| IBIS file generated by GenIBIS.pl Version 3.22
|   dm385
[IBIS ver]   4.1
[File name]   dm385.ibs
[File Rev]   3.0
[Date]   Tue Oct 30, 2012, 8:51:53
[Source]   Data created at Texas Instruments
[Notes]   CHECKED BY IBISCK4.
   166 warnings can be ignored
   Some pins may contain selectors which are not valid options
   for that particular pin.
   Please refer to the device datasheet for information on picking
   the correct selector model, which depends on various software
   register configurations.
   Some pins are modeled as IO or tri-state for output mode.
[Disclaimer] Please be aware that in the absence of a written agreement,
   Texas Instruments (TI) assumes no liability for: 1) the
   accuracy of the IBIS models provided to your company, 2) the
   proper functioning of these IBIS models in your design or for
   any resulting applications, or, 3) infringement of patents,
   copyrights, or intellectual property rights resulting from
   your use of these IBIS models. TI provides IBIS models as a
   service to our customers and therefore reserves the right to
   limit distribution of the IBIS models.
[Copyright]   Property of Texas Instruments Incorporated. Unauthorised
   reproduction and/or distribution is strictly prohibited. This
   product is protected under copyright law and trade secret law
   as an unpublished work. Created 2010,(C) Copyright 2010,
   Texas Instruments Incorporated., All Rights Reserved. These
   commodities are under the U.S. Government distribution license
   control.As such,they are not to be re-exported without the
   prior approval of the U.S. Department of Commerce.
|   Component dm385
[Component]   dm385
[Manufacturer]   Texas Instruments.
| Source IO level model revisions
|Model   Revision   Date
|BC1833DV40DCPBFBP18LL_SSDHH   1.1   May 27, 2010
|IQ1833DVTCKPBFBP18LL_SSDHH   1.1   May 27, 2010
|BC1833DV50BPBFBP18LL_SSDHV   1.1   May 30, 2010
|IHHV1833DVHYP18LL_SSDHH   1.1   May 27, 2010
|BC1833DV50BPBFBP18LL_SSDHH   1.1   May 30, 2010
|BI2C1833DVFZP18_SSDHH   1.0   May 28, 2010
|BC1833DV40DCPBFBP18LL_SSDHV   1.1   May 27, 2010
|BCSHTLTCSCDVPBFZ_SSDHV   1.0   May 31, 2010
|BCSHTLTCSCDDVPBFZ_SSDHV   1.0   May 31, 2010
[Package]
|   typ   min   max
R_pkg   0.227048417721519   2.87E-2   6.12E-1
L_pkg   1.80481962025317E-009 3.33E-10   4.72E-9
C_pkg   8.93439873417721E-013 5.09E-13   1.66E-12
[Pin]   signal_name   model_name   R_pin   L_pin   C_pin
AF27   AUD_CLKIN1   Selector_5   1.66E-1   1.31E-9   7.51E-13
AG30   AUD_CLKIN2   Selector_5   2.51E-1   2.00E-9   7.85E-13
AF31   AUD_CLKIN0   Selector_5   2.58E-1   2.21E-9   7.02E-13
V30   AUXOSC_MXI   NC
U31   AUXOSC_MXO   NC
AJ31   CLKIN32   Selector_5   3.03E-1   2.21E-9   6.52E-13
AA2   CSI2_DX[2]   NC
V2   CSI2_DY[4]   NC
AC2   CSI2_DY[0]   NC
Y2   CSI2_DY[2]   NC
W2   CSI2_DX[3]   NC
V1   CSI2_DX[4]   NC
W1   CSI2_DY[3]   NC
AA1   CSI2_DX[1]   NC
AB2   CSI2_DX[0]   NC
AB1   CSI2_DY[1]   NC
AL26   DDR[0]_WEN   Selector_9   3.09E-1   2.24E-9   7.45E-13
AJ27   DDR[0]_A[3]   Selector_9   3.09E-1   2.18E-9   9.15E-13
AL23   DDR[0]_A[14]   Selector_9   3.06E-1   2.10E-9   8.49E-13
AK24   DDR[0]_A[11]   Selector_9   3.08E-1   2.21E-9   7.45E-13
AG23   DDR[0]_A[7]   Selector_9   2.86E-1   1.99E-9   1.03E-12
AK9   DDR[0]_D[1]   Selector_8   2.35E-1   1.65E-9   8.84E-13
AJ15   DDR[0]_DQM[2]   Selector_9   2.37E-1   1.45E-9   7.37E-13
AK30   DDR[0]_A[6]   Selector_9   3.09E-1   2.37E-9   8.54E-13
AH23   DDR[0]_A[12]   Selector_9   2.98E-1   2.05E-9   8.52E-13
AL27   DDR[0]_CLK   Selector_9   2.52E-1   2.04E-9   8.22E-13
AH19   DDR[0]_D[26]   Selector_8   2.46E-1   1.65E-9   1.02E-12
AG20   DDR[0]_D[31]   Selector_8   2.57E-1   1.66E-9   1.01E-12
AK29   DDR[0]_A[9]   Selector_9   3.11E-1   2.17E-9   7.34E-13
AC19   DDR[0]_D[29]   Selector_8   1.65E-1   6.79E-10   1.25E-12
AK14   DDR[0]_D[15]   Selector_8   2.56E-1   1.50E-9   8.22E-13
AK13   DDR[0]_D[12]   Selector_8   2.59E-1   1.57E-9   7.06E-13
AK17   DDR[0]_DQS[2]N   Selector_12  2.03E-1   1.95E-9   7.17E-13
AG16   DDR[0]_D[21]   Selector_8   2.33E-1   1.25E-9   8.85E-13
AD15   DDR[0]_D[18]   Selector_8   1.61E-1   1.07E-9   1.03E-12
AC16   DDR[0]_D[23]   Selector_8   1.58E-1   8.32E-10   1.14E-12
AJ23   DDR[0]_A[2]   Selector_9   3.05E-1   2.12E-9   9.93E-13
AL15   DDR[0]_DQS[1]   Selector_12  2.28E-1   1.81E-9   6.85E-13
AG12   DDR[0]_D[9]   Selector_8   2.59E-1   1.32E-9   6.94E-13
AD19   DDR[0]_D[28]   Selector_8   1.70E-1   1.29E-9   1.05E-12
AK15   DDR[0]_DQS[1]N   Selector_12  2.25E-1   1.76E-9   9.52E-13
AJ12   DDR[0]_D[8]   Selector_8   2.60E-1   1.53E-9   8.05E-13
AD12   DDR[0]_D[10]   Selector_8   1.72E-1   7.55E-10   1.03E-12
AL8   DDR[0]_DQM[0]   Selector_9   2.41E-1   1.77E-9   7.77E-13
AJ16   DDR[0]_D[20]   Selector_8   2.33E-1   1.47E-9   7.48E-13
AL12   DDR[0]_D[7]   Selector_8   2.40E-1   1.76E-9   6.73E-13
AL30   DDR[0]_VTP   NC
AL21   DDR[0]_ODT[0]   Selector_9   2.99E-1   2.04E-9   7.45E-13
AL24   DDR[0]_A[0]   Selector_9   3.06E-1   2.36E-9   8.02E-13
AF19   DDR[0]_D[27]   Selector_8   2.32E-1   1.51E-9   9.24E-13
AL20   DDR[0]_DQS[3]   Selector_12  2.23E-1   2.10E-9   8.50E-13
AK22   DDR[0]_A[15]   Selector_9   2.99E-1   2.06E-9   8.71E-13
AK26   DDR[0]_BA[0]   Selector_9   2.88E-1   2.01E-9   8.71E-13
AJ19   DDR[0]_D[25]   Selector_8   2.48E-1   1.87E-9   8.59E-13
AH27   DDR[0]_A[5]   Selector_9   2.90E-1   2.10E-9   8.89E-13
AK25   DDR[0]_CASN   Selector_9   3.10E-1   2.38E-9   8.70E-13
AJ20   DDR[0]_D[30]   Selector_8   2.58E-1   1.54E-9   8.11E-13
AK10   DDR[0]_D[2]   Selector_8   2.34E-1   1.55E-9   7.39E-13
AD23   DDR[0]_A[10]   Selector_9   1.90E-1   1.33E-9   1.10E-12
AD16   DDR[0]_D[22]   Selector_8   1.53E-1   7.63E-10   1.20E-12
AK20   DDR[0]_DQS[3]N   Selector_12  2.20E-1   1.71E-9   7.20E-13
AK16   DDR[0]_D[19]   Selector_8   2.34E-1   2.09E-9   7.88E-13
AJ25   DDR[0]_RASN   Selector_9   3.06E-1   2.36E-9   1.10E-12
AH11   DDR[0]_D[4]   Selector_8   2.36E-1   1.63E-9   1.09E-12
AL14   DDR[0]_D[14]   Selector_8   2.77E-1   2.19E-9   7.20E-13
AL9   DDR[0]_D[0]   Selector_8   2.41E-1   1.84E-9   6.60E-13
AK19   DDR[0]_D[24]   Selector_8   2.63E-1   1.99E-9   8.03E-13
AK27   DDR[0]_CLKN   Selector_9   2.55E-1   1.99E-9   7.91E-13
AJ11   DDR[0]_D[3]   Selector_8   2.28E-1   1.48E-9   7.79E-13
AC22   DDR[0]_A[1]   Selector_9   1.99E-1   1.56E-9   1.21E-12
AK28   DDR[0]_A[4]   Selector_9   3.07E-1   2.35E-9   9.20E-13
AF23   DDR[0]_BA[1]   Selector_9   2.79E-1   1.74E-9   9.46E-13
AK18   DDR[0]_DQM[3]   Selector_9   2.62E-1   1.71E-9   7.74E-13
AK11   DDR[0]_DQS[0]N   Selector_12  1.97E-1   1.57E-9   7.59E-13
AK12   DDR[0]_DQM[1]   Selector_9   2.61E-1   1.73E-9   6.87E-13
AB21   DDR[0]_CS[0]N   Selector_9   1.89E-1   1.60E-9   1.21E-12
AH15   DDR[0]_D[16]   Selector_8   2.32E-1   1.43E-9   7.75E-13
AL17   DDR[0]_DQS[2]   Selector_12  2.06E-1   2.04E-9   6.57E-13
AF15   DDR[0]_D[17]   Selector_8   2.33E-1   1.25E-9   7.62E-13
AD9   DDR[0]_D[5]   Selector_8   1.50E-1   1.11E-9   1.08E-12
AF11   DDR[0]_D[6]   Selector_8   2.23E-1   1.41E-9   7.17E-13
AL29   DDR[0]_A[8]   Selector_9   3.11E-1   2.25E-9   8.11E-13
AC13   DDR[0]_D[13]   Selector_8   1.77E-1   9.38E-10   7.90E-13
AA20   DDR[0]_RST   Selector_9   1.14E-1   1.28E-9   1.23E-12
AD20   DDR[0]_CKE   Selector_9   1.85E-1   1.25E-9   1.14E-12
AL11   DDR[0]_DQS[0]   Selector_12  2.00E-1   1.74E-9   8.08E-13
AK23   DDR[0]_A[13]   Selector_9   3.07E-1   2.17E-9   9.86E-13
AH25   DDR[0]_BA[2]   Selector_9   2.98E-1   2.18E-9   1.24E-12
AB12   DDR[0]_D[11]   Selector_8   1.92E-1   9.34E-10   1.25E-12
F30   DEVOSC_MXI   NC
G31   DEVOSC_MXO   NC
U28   DEVOSC_WAKE   Selector_5   1.35E-1   1.20E-9   7.62E-13
AH1   EMAC[0]_MCOL   Selector_5   3.85E-1   2.94E-9   9.55E-13
AL3   EMAC[0]_MRXD[2]   Selector_5   3.82E-1   2.76E-9   1.06E-12
AH8   EMAC[0]_MTXD[6]   Selector_5   1.63E-1   1.30E-9   7.04E-13
AJ6   EMAC[0]_MRXDV   Selector_5   2.42E-1   1.83E-9   7.69E-13
AJ2   EMAC[0]_MRXER   Selector_5   3.56E-1   2.48E-9   9.44E-13
AE4   EMAC[0]_MTXD[3]   Selector_5   1.06E-1   1.05E-9   9.05E-13
AG1   EMAC_RMREFCLK   Selector_5   3.61E-1   2.77E-9   1.09E-12
AK7   EMAC[0]_MTXD[2]   Selector_5   2.54E-1   2.10E-9   9.24E-13
AL5   EMAC[0]_MRXD[6]   Selector_5   3.30E-1   2.32E-9   9.10E-13
AK4   EMAC[0]_MRXD[4]   Selector_5   3.22E-1   2.36E-9   1.06E-12
AK3   EMAC[0]_MRXD[3]   Selector_5   3.32E-1   2.46E-9   1.18E-12
AK6   EMAC[0]_MTXD[0]   Selector_5   2.62E-1   2.01E-9   9.37E-13
AL6   EMAC[0]_GMTCLK   Selector_5   3.33E-1   2.48E-9   9.02E-13
AJ7   EMAC[0]_MTXD[1]   Selector_5   2.29E-1   1.79E-9   9.75E-13
AK5   EMAC[0]_MRXD[7]   Selector_5   2.92E-1   2.07E-9   1.01E-12
AJ8   EMAC[0]_MTXD[5]   Selector_5   2.05E-1   1.57E-9   7.51E-13
AF8   EMAC[0]_MTXEN   Selector_5   4.94E-2   5.14E-10   6.62E-13
AH2   EMAC[0]_MCRS   Selector_5   3.49E-1   2.48E-9   1.18E-12
AG4   EMAC[0]_MTCLK   Selector_5   2.64E-1   1.97E-9   1.04E-12
AK1   EMAC[0]_MRCLK   Selector_5   4.24E-1   2.94E-9   1.10E-12
AK8   EMAC[0]_MTXD[4]   Selector_5   2.39E-1   1.84E-9   9.63E-13
AL2   EMAC[0]_MRXD[1]   Selector_5   4.00E-1   2.78E-9   1.05E-12
AG8   EMAC[0]_MTXD[7]   Selector_5   9.95E-2   7.49E-10   7.36E-13
AJ4   EMAC[0]_MRXD[5]   Selector_5   2.84E-1   2.10E-9   9.81E-13
AK2   EMAC[0]_MRXD[0]   Selector_5   3.75E-1   2.65E-9   1.01E-12
A18   EMU0   Selector_16  2.53E-1   2.14E-9   6.98E-13
B19   EMU1   Selector_16  2.48E-1   1.95E-9   8.34E-13
R2   GPMC_D[13]   Selector_5   2.29E-1   1.71E-9   5.72E-13
AA10   GPMC_ADVN_ALE   Selector_5   1.88E-1   1.72E-9   1.00E-12
M2   GPMC_A[17]   Selector_5   2.33E-1   1.87E-9   7.47E-13
M1   GPMC_A[16]   Selector_5   2.62E-1   2.35E-9   5.77E-13
M3   GPMC_A[18]   Selector_5   2.04E-1   1.56E-9   8.46E-13
T8   GPMC_D[9]   Selector_5   4.04E-2   4.40E-10   7.71E-13
T1   GPMC_D[8]   Selector_5   2.67E-1   2.02E-9   6.50E-13
W6   GPMC_D[0]   Selector_5   1.30E-1   1.38E-9   1.04E-12
N9   GPMC_A[20]   Selector_5   3.84E-2   4.90E-10   7.79E-13
M5   GPMC_A[19]   Selector_5   1.34E-1   1.21E-9   7.39E-13
T3   GPMC_D[6]   Selector_5   1.90E-1   1.37E-9   7.92E-13
W9   GPMC_D[4]   Selector_5   9.55E-2   1.25E-9   1.07E-12
N1   GPMC_A[21]   Selector_5   2.61E-1   1.95E-9   5.85E-13
AB9   GPMC_CLK   Selector_5   2.06E-1   1.80E-9   1.13E-12
N2   GPMC_A[22]   Selector_5   2.29E-1   1.70E-9   7.54E-13
Y5   GPMC_WEN   Selector_5   1.86E-1   1.70E-9   1.05E-12
R1   GPMC_D[14]   Selector_5   2.65E-1   1.82E-9   6.57E-13
R6   GPMC_D[10]   Selector_5   9.06E-2   7.90E-10   7.40E-13
W8   GPMC_WAIT[0]   Selector_5   7.07E-2   9.84E-10   1.05E-12
Y3   GPMC_BE[0]N_CLE   Selector_5   2.26E-1   2.44E-9   8.93E-13
AC9   GPMC_CS[0]N   Selector_5   2.25E-1   1.92E-9   1.34E-12
P2   GPMC_D[15]   Selector_5   2.07E-1   1.56E-9   6.41E-13
W4   GPMC_D[1]   Selector_5   1.69E-1   1.62E-9   8.93E-13
Y8   GPMC_OE_REN   Selector_5   8.78E-2   1.18E-9   1.09E-12
AC3   GPMC_CS[2]N   Selector_5   2.27E-1   1.79E-9   7.80E-13
T5   GPMC_D[5]   Selector_5   1.08E-1   1.05E-9   7.69E-13
AG6   GPMC_CS[4]N   Selector_5   2.47E-1   2.00E-9   1.10E-12
W3   GPMC_D[2]   Selector_5   2.21E-1   1.94E-9   8.39E-13
R3   GPMC_D[12]   Selector_5   1.81E-1   1.43E-9   6.41E-13
AA12   GPMC_CS[1]N   Selector_5   1.16E-1   1.42E-9   1.27E-12
T2   GPMC_D[7]   Selector_5   2.27E-1   1.73E-9   6.57E-13
AF2   GPMC_CS[3]N   Selector_5   3.08E-1   2.32E-9   9.30E-13
R8   GPMC_A[23]   Selector_5   3.63E-2   3.74E-10   7.91E-13
U2   GPMC_D[3]   Selector_5   2.06E-1   1.77E-9   8.63E-13
Y11   GPMC_BE[1]N   Selector_5   1.65E-1   1.70E-9   1.27E-12
R4   GPMC_D[11]   Selector_5   1.33E-1   1.15E-9   7.09E-13
A9   HDDAC_A   NC
B7   HDDAC_VREF   NC
B6   HDDAC_IREF   NC
E9   HDDAC_HSYNC   Selector_4   6.43E-2   5.68E-10   6.01E-13
A8   HDDAC_B   NC
D9   HDDAC_VSYNC   Selector_4   9.70E-2   9.00E-10   8.07E-13
B8   HDDAC_C   NC
A15   HDMI_CLKP   NC
A12   HDMI_DN2   NC
B13   HDMI_DN1   NC
A14   HDMI_DN0   NC
B14   HDMI_DP0   NC
B15   HDMI_CLKN   NC
A11   HDMI_DP2   NC
B12   HDMI_DP1   NC
D2   I2C[1]_SCL   Selector_2   3.52E-1   2.57E-9   1.14E-12
T24   I2C[0]_SDA   Selector_2   3.75E-2   3.33E-10   9.91E-13
T27   I2C[0]_SCL   Selector_2   1.10E-1   9.87E-10   6.35E-13
D1   I2C[1]_SDA   Selector_2   3.78E-1   2.72E-9   8.43E-13
Y21   MCA[1]_AXR[1]   Selector_14  8.08E-2   9.66E-10   1.38E-12
AC24   MCA[1]_AFSR   Selector_14  5.51E-2   6.17E-10   8.58E-13
AD29   MCA[1]_ACLKR   Selector_14  1.99E-1   1.54E-9   7.47E-13
AD30   MCA[0]_ACLKR   Selector_14  2.42E-1   1.99E-9   6.99E-13
AF29   MCA[0]_AXR[0]   Selector_14  2.04E-1   1.55E-9   6.97E-13
AC31   MCA[0]_AXR[3]   Selector_14  2.55E-1   1.97E-9   7.06E-13
AE31   MCA[0]_AXR[1]   Selector_14  2.49E-1   1.80E-9   6.83E-13
Y22   MCA[1]_AXR[0]   Selector_14  4.32E-2   7.12E-10   9.06E-13
AC23   MCA[1]_ACLKX   Selector_14  6.51E-2   7.77E-10   9.32E-13
AD27   MCA[0]_AXR[5]   Selector_14  1.30E-1   1.24E-9   8.34E-13
AD28   MCA[0]_ACLKX   Selector_14  1.42E-1   1.50E-9   6.83E-13
AD26   MCA[0]_AXR[4]   Selector_14  1.05E-1   1.03E-9   7.96E-13
AE30   MCA[0]_AXR[2]   Selector_14  2.22E-1   1.81E-9   7.42E-13
AB22   MCA[1]_AFSX   Selector_14  5.70E-2   5.46E-10   9.60E-13
AE29   MCA[0]_AFSX   Selector_14  1.74E-1   1.70E-9   7.57E-13
AF30   MCA[0]_AFSR   Selector_14  2.24E-1   1.87E-9   7.37E-13
AG2   MDCLK   Selector_5   3.17E-1   2.33E-9   9.92E-13
AG3   MDIO   Selector_5   2.95E-1   2.33E-9   8.47E-13
AH31   NMIN   Selector_7   3.08E-1   2.07E-9   8.90E-13
K31   PCIE_TXN0   NC
K30   PCIE_RXP0   NC
L31   PCIE_TXP0   NC
J30   PCIE_RXN0   NC
AH30   PORN   Selector_6   2.59E-1   1.86E-9   9.14E-13
AH29   RESETN   Selector_7   2.35E-1   1.62E-9   6.89E-13
AJ30   RSTOUT_WD_OUTN   Selector_10  2.70E-1   1.93E-9   9.49E-13
J25   RSV0   NC
H24   RSV2   NC
H28   RSV3   NC
L30   RSV27   NC
M30   RSV28   NC
N30   RSV29   NC
N31   RSV30   NC
P31   RSV31   NC
R30   RSV32   NC
T30   RSV33   NC
AK21   RSV42   Selector_9   2.98E-1   1.94E-9   9.19E-13
P30   RSV43   NC
N29   RTCK   Selector_13  1.55E-1   1.58E-9   8.66E-13
AB31   SD0_DAT[6]   Selector_14  2.34E-1   1.97E-9   7.86E-13
AC30   SD0_DAT[7]   Selector_14  2.32E-1   1.88E-9   8.26E-13
AB30   SD0_CLK   Selector_5   2.14E-1   1.76E-9   6.98E-13
Y30   SD0_DAT[3]   Selector_5   1.93E-1   1.62E-9   7.33E-13
AA28   SD0_DAT[0]   Selector_5   1.42E-1   1.34E-9   7.40E-13
AA26   SD0_DAT[1]_SDIRQN   Selector_5   9.56E-2   1.03E-9   8.42E-13
Y31   SD0_DAT[2]_SDRWN   Selector_5   2.25E-1   1.96E-9   7.06E-13
AA29   SD0_CMD   Selector_5   1.70E-1   1.55E-9   7.83E-13
AA30   SD1_DAT[1]_SDIRQN   Selector_5   2.74E-1   2.10E-9   8.23E-13
W31   SD1_DAT[0]   Selector_5   2.51E-1   1.84E-9   7.39E-13
W30   SD1_CLK   Selector_4   2.00E-1   1.61E-9   7.96E-13
Y27   SD1_DAT[3]   Selector_5   1.24E-1   1.16E-9   8.87E-13
Y29   SD1_CMD   Selector_5   1.83E-1   1.49E-9   8.27E-13
U29   SD1_DAT[2]_SDRWN   Selector_5   1.62E-1   1.41E-9   6.87E-13
AE3   SD2_DAT[7]   Selector_5   2.41E-1   1.84E-9   9.36E-13
AC6   SD2_SCLK   Selector_5   1.65E-1   1.48E-9   8.89E-13
AC8   SD2_DAT[2]_SDRWN   Selector_5   1.27E-1   1.10E-9   1.08E-12
AC4   SD2_DAT[0]   Selector_5   1.93E-1   1.54E-9   7.61E-13
AC5   SD2_DAT[1]_SDIRQN   Selector_5   1.79E-1   1.54E-9   8.62E-13
AD2   SD2_DAT[4]   Selector_5   2.68E-1   2.16E-9   9.23E-13
AD1   SD2_DAT[3]   Selector_5   3.11E-1   2.59E-9   6.39E-13
AE2   SD2_DAT[6]   Selector_5   2.66E-1   2.13E-9   6.74E-13
AE1   SD2_DAT[5]   Selector_5   3.04E-1   2.41E-9   8.36E-13
H31   SERDES_CLKN   NC
H30   SERDES_CLKP   NC
N23   SPI[1]_D[0]   Selector_11  6.99E-2   6.82E-10   1.09E-12
J28   SPI[0]_D[0]   Selector_11  1.42E-1   1.36E-9   8.74E-13
M29   SPI[1]_SCLK   Selector_11  1.51E-1   1.45E-9   8.33E-13
N24   SPI[0]_SCLK   Selector_16  1.14E-1   1.30E-9   1.22E-12
G28   SPI[0]_SCS[1]N   Selector_11  1.77E-1   1.43E-9   7.49E-13
J27   SPI[0]_D[1]   Selector_11  1.16E-1   1.07E-9   6.17E-13
J29   SPI[1]_SCS[0]N   Selector_11  1.53E-1   1.56E-9   6.76E-13
G29   SPI[0]_SCS[0]N   Selector_11  1.88E-1   1.53E-9   7.64E-13
M27   SPI[1]_D[1]   Selector_11  9.96E-2   1.02E-9   7.76E-13
T29   TCLK   Selector_15  1.55E-1   1.39E-9   7.00E-13
N28   TDI   Selector_3   1.49E-1   1.31E-9   8.10E-13
U26   TDO   Selector_4   8.14E-2   8.38E-10   6.47E-13
T31   TMS   Selector_7   2.63E-1   2.02E-9   6.65E-13
U24   TRSTN   Selector_7   3.68E-2   3.94E-10   7.07E-13
B10   TV_VFB0   NC
B11   TV_RSET   NC
B9   TV_OUT0   NC
E30   UART0_DTRN   Selector_11  2.32E-1   1.69E-9   7.42E-13
J26   UART0_RXD   Selector_3   5.32E-2   5.77E-10   6.66E-13
E29   UART0_DSRN   Selector_11  2.20E-1   1.69E-9   7.10E-13
E28   UART0_TXD   Selector_1   1.93E-1   1.74E-9   9.07E-13
N26   UART0_RIN   Selector_11  1.22E-1   1.26E-9   7.65E-13
D31   UART0_RTSN   Selector_11  2.94E-1   2.30E-9   9.20E-13
D30   UART0_CTSN   Selector_11  2.65E-1   2.20E-9   8.68E-13
E31   UART0_DCDN   Selector_11  2.75E-1   2.23E-9   8.81E-13
L22   UART2_RXD   Selector_11  1.11E-1   1.13E-9   1.58E-12
M21   UART2_TXD   Selector_11  1.42E-1   1.48E-9   1.66E-12
A21   USB0_DP   NC
A20   USB0_ID   NC
B22   USB0_VBUSIN   NC
B20   USB0_CE   NC
B21   USB0_DM   NC
K23   USB0_DRVVBUS   Selector_11  1.02E-1   1.05E-9   1.20E-12
A23   USB1_DP   NC
A24   USB1_ID   NC
C21   USB1_CE   NC
B24   USB1_VBUSIN   NC
B23   USB1_DM   NC
D17   VIN[0]A_D[4]   Selector_11  1.46E-1   1.34E-9   7.23E-13
H16   VIN[0]A_D[13]_BD[5]  Selector_16  4.14E-2   5.78E-10   8.16E-13
L20   VIN[0]A_D[6]   Selector_11  2.11E-1   1.81E-9   1.09E-12
D13   VIN[0]A_HSYNC   Selector_11  1.73E-1   1.98E-9   8.59E-13
C9   VIN[0]A_CLK   Selector_11  1.40E-1   1.69E-9   7.74E-13
K11   VIN[0]A_D[16]   Selector_5   1.34E-1   1.26E-9   1.25E-12
B18   VIN[0]A_D[0]   Selector_11  2.31E-1   1.90E-9   7.19E-13
B16   VIN[0]A_D[8]_BD[0]   Selector_11  2.10E-1   1.77E-9   5.77E-13
B5   VIN[0]A_DE1   Selector_5   2.78E-1   1.92E-9   8.57E-13
A6   VIN[0]A_D[22]   Selector_5   2.74E-1   2.02E-9   6.72E-13
C13   VIN[0]A_VSYNC   Selector_11  2.01E-1   2.09E-9   8.83E-13
J16   VIN[0]A_D[12]_BD[4]  Selector_16  4.57E-2   8.08E-10   9.63E-13
H20   VIN[0]A_D[7]   Selector_11  1.44E-1   1.76E-9   1.03E-12
F17   VIN[0]A_D[5]   Selector_11  7.66E-2   8.46E-10   8.35E-13
A17   VIN[0]A_D[1]   Selector_11  2.54E-1   2.21E-9   5.62E-13
F13   VIN[0]A_D[14]_BD[6]  Selector_16  1.19E-1   1.18E-9   7.73E-13
C7   VIN[0]A_D[21]   Selector_5   1.72E-1   1.61E-9   7.09E-13
C12   VIN[0]A_DE   Selector_16  1.85E-1   1.77E-9   7.90E-13
H13   VIN[0]A_D[15]_BD[7]  Selector_16  3.45E-2   5.26E-10   1.05E-12
K10   VIN[0]A_D[18]   Selector_5   1.04E-1   1.29E-9   1.15E-12
H12   VIN[0]B_CLK   Selector_16  9.56E-2   7.63E-10   9.70E-13
E12   VIN[0]A_D[17]   Selector_5   1.39E-1   1.57E-9   8.57E-13
C16   VIN[0]A_D[9]_BD[1]   Selector_16  1.76E-1   1.36E-9   6.41E-13
F9   VIN[0]A_D[20]   Selector_5   5.09E-2   5.93E-10   6.53E-13
E16   VIN[0]A_D[10]_BD[2]  Selector_16  1.07E-1   9.58E-10   7.96E-13
C17   VIN[0]A_D[3]   Selector_11  1.94E-1   1.67E-9   7.64E-13
H17   VIN[0]A_D[11]_BD[3]  Selector_16  6.05E-2   7.18E-10   9.63E-13
J13   VIN[0]A_FLD   Selector_16  1.19E-1   1.15E-9   9.81E-13
A5   VIN[0]A_D[23]   Selector_5   2.65E-1   1.94E-9   8.01E-13
B17   VIN[0]A_D[2]   Selector_11  2.09E-1   1.89E-9   6.48E-13
D7   VIN[0]A_D[19]   Selector_5   1.24E-1   1.23E-9   7.02E-13
A3   VIN[0]B_FLD   Selector_5   3.26E-1   2.44E-9   9.24E-13
C5   VIN[0]B_DE   Selector_5   2.54E-1   1.79E-9   8.45E-13
B4   VIN[0]A_FLD1   Selector_5   2.78E-1   1.97E-9   8.74E-13
L3   VOUT[1]_G_Y_YC[8]   Selector_5   1.66E-1   1.32E-9   7.96E-13
B27   VOUT[0]_G_Y_YC[8]   Selector_13  4.86E-1   4.13E-9   1.00E-12
C25   VOUT[0]_G_Y_YC[2]   Selector_16  4.92E-1   4.09E-9   1.09E-12
L2   VOUT[1]_G_Y_YC[2]   Selector_5   2.34E-1   1.94E-9   7.55E-13
D5   VOUT[1]_B_CB_C[1]   Selector_5   2.40E-1   1.73E-9   8.85E-13
J1   VOUT[1]_G_Y_YC[5]   Selector_5   3.03E-1   2.19E-9   6.15E-13
E2   VOUT[1]_HSYNC   Selector_5   3.24E-1   2.34E-9   7.87E-13
K2   VOUT[1]_R_CR[9]   Selector_5   2.39E-1   1.90E-9   8.14E-13
B25   VOUT[0]_G_Y_YC[7]   Selector_13  4.43E-1   3.16E-9   1.06E-12
B3   VOUT[0]_FLD   Selector_5   3.12E-1   2.30E-9   9.13E-13
D21   VOUT[0]_B_CB_C[3]   Selector_16  2.22E-1   2.02E-9   9.46E-13
B28   VOUT[0]_R_CR[3]   Selector_16  5.48E-1   4.52E-9   1.20E-12
F21   VOUT[0]_HSYNC   Selector_13  1.58E-1   1.50E-9   1.09E-12
H6   VOUT[1]_G_Y_YC[3]   Selector_5   1.73E-1   1.53E-9   8.12E-13
J10   VOUT[1]_FLD   Selector_5   4.39E-2   7.65E-10   1.05E-12
F24   VOUT[0]_B_CB_C[2]   Selector_16  2.33E-1   2.01E-9   1.10E-12
A26   VOUT[0]_G_Y_YC[6]   Selector_13  4.67E-1   3.58E-9   1.07E-12
J2   VOUT[1]_R_CR[8]   Selector_5   2.25E-1   1.83E-9   7.52E-13
G1   VOUT[1]_B_CB_C[5]   Selector_5   3.30E-1   2.54E-9   8.23E-13
K22   VOUT[0]_CLK   Selector_13  1.58E-1   2.10E-9   1.06E-12
L4   VOUT[1]_R_CR[3]   Selector_5   1.64E-1   1.39E-9   5.09E-13
E24   VOUT[0]_B_CB_C[7]   Selector_13  2.56E-1   2.41E-9   1.19E-12
L6   VOUT[1]_R_CR[2]   Selector_5   8.86E-2   9.28E-10   8.58E-13
L12   VOUT[1]_R_CR[6]   Selector_5   6.32E-2   9.24E-10   1.37E-12
A30   VOUT[0]_R_CR[8]   Selector_13  6.12E-1   4.47E-9   1.23E-12
B29   VOUT[0]_R_CR[4]   Selector_13  5.47E-1   3.88E-9   1.38E-12
J9   VOUT[1]_G_Y_YC[7]   Selector_5   1.45E-1   1.37E-9   1.11E-12
C20   VOUT[0]_AVID   Selector_16  2.07E-1   2.09E-9   7.79E-13
H3   VOUT[1]_B_CB_C[7]   Selector_5   2.41E-1   1.81E-9   9.03E-13
C26   VOUT[0]_G_Y_YC[3]   Selector_16  5.42E-1   4.48E-9   1.33E-12
M11   VOUT[1]_R_CR[5]   Selector_5   6.82E-2   9.06E-10   1.32E-12
J23   VOUT[0]_B_CB_C[4]   Selector_13  1.55E-1   1.92E-9   1.32E-12
H9   VOUT[1]_B_CB_C[0]   Selector_5   6.96E-2   8.39E-10   7.72E-13
H2   VOUT[1]_R_CR[4]   Selector_5   3.39E-1   2.98E-9   8.40E-13
B26   VOUT[0]_G_Y_YC[5]   Selector_13  4.86E-1   3.78E-9   1.23E-12
E26   VOUT[0]_G_Y_YC[4]   Selector_13  5.53E-1   4.72E-9   1.56E-12
B31   VOUT[0]_R_CR[9]   Selector_13  6.11E-1   4.51E-9   1.27E-12
A29   VOUT[0]_R_CR[5]   Selector_13  5.79E-1   4.17E-9   1.15E-12
A27   VOUT[0]_G_Y_YC[9]   Selector_13  5.11E-1   4.30E-9   1.04E-12
J8   VOUT[1]_G_Y_YC[4]   Selector_5   1.17E-1   1.09E-9   6.74E-13
D24   VOUT[0]_B_CB_C[8]   Selector_13  2.72E-1   2.61E-9   1.22E-12
C30   VOUT[0]_R_CR[6]   Selector_13  5.56E-1   4.08E-9   1.51E-12
C2   VOUT[1]_R_CR[0]   Selector_5   3.73E-1   2.49E-9   9.34E-13
F3   VOUT[1]_B_CB_C[4]   Selector_5   2.86E-1   2.02E-9   8.63E-13
J24   VOUT[0]_B_CB_C[6]   Selector_13  2.73E-1   2.62E-9   1.30E-12
G2   VOUT[1]_B_CB_C[6]   Selector_5   2.99E-1   2.35E-9   7.67E-13
F5   VOUT[1]_VSYNC   Selector_5   2.31E-1   1.67E-9   1.03E-12
C24   VOUT[0]_B_CB_C[9]   Selector_13  2.95E-1   2.80E-9   1.02E-12
H5   VOUT[1]_B_CB_C[9]   Selector_5   2.12E-1   1.73E-9   1.03E-12
M8   VOUT[1]_B_CB_C[2]   Selector_5   2.87E-2   4.25E-10   7.42E-13
C28   VOUT[0]_R_CR[2]   Selector_16  5.31E-1   3.97E-9   1.39E-12
G3   VOUT[1]_B_CB_C[8]   Selector_5   2.72E-1   2.26E-9   8.65E-13
B30   VOUT[0]_R_CR[7]   Selector_13  5.89E-1   4.20E-9   1.37E-12
F2   VOUT[1]_B_CB_C[3]   Selector_5   3.10E-1   2.28E-9   9.84E-13
F1   VOUT[1]_AVID   Selector_5   3.29E-1   2.44E-9   7.25E-13
A2   VOUT[1]_G_Y_YC[1]   Selector_5   3.72E-1   2.89E-9   9.50E-13
C1   VOUT[1]_R_CR[1]   Selector_5   3.93E-1   2.74E-9   8.47E-13
B2   VOUT[1]_G_Y_YC[0]   Selector_5   3.58E-1   2.54E-9   1.08E-12
H23   VOUT[0]_B_CB_C[5]   Selector_13  1.44E-1   1.58E-9   9.40E-13
K1   VOUT[1]_G_Y_YC[9]   Selector_5   2.77E-1   2.16E-9   7.40E-13
H4   VOUT[1]_G_Y_YC[6]   Selector_5   2.16E-1   1.61E-9   9.62E-13
E20   VOUT[0]_VSYNC   Selector_13  1.60E-1   1.53E-9   1.02E-12
M10   VOUT[1]_R_CR[7]   Selector_5   4.38E-2   5.27E-10   7.99E-13
D3   VOUT[1]_CLK   Selector_5   3.17E-1   2.20E-9   6.90E-13
AL18   VREFSSTL_DDR[0]   NC
U30   VSSA_AUXOSC   NC
G30   VSSA_DEVOSC   NC
[Diff Pin]   inv_pin   vdiff   tdelay_typ
|DDR[0]_DQS[3]   DDR[0]_DQS[3]N
AL20   AK20   200m   NA
|DDR[0]_DQS[2]   DDR[0]_DQS[2]N
AL17   AK17   200m   NA
|DDR[0]_DQS[1]   DDR[0]_DQS[1]N
AL15   AK15   200m   NA
|DDR[0]_DQS[0]   DDR[0]_DQS[0]N
AL11   AK11   200m   NA
|   Usage OUTPUT#1.8/3.3#X#X#BC1833DV50BPBFBP18LL_SSDHV.PAD
|   Base model BC1833DV50BPBFBP18LL_SSDHV
[Model Selector] Selector_1
Model_37 I/O,1.8V,Pull-down,NORMAL,IND,5%
Model_38 I/O,1.8V,Pull-up,NORMAL,IND,5%
Model_39 I/O,1.8V,Pull-up/down off,NORMAL,IND,5%
Model_40 I/O,3.3V,Pull-down,NORMAL,IND,5%
Model_41 I/O,3.3V,Pull-up,NORMAL,IND,5%
Model_42 I/O,3.3V,Pull-up/down off,NORMAL,IND,5%
Model_43 I/O,1.8V,Pull-down,NORMAL,IND,10%
Model_44 I/O,1.8V,Pull-up,NORMAL,IND,10%
Model_45 I/O,1.8V,Pull-up/down off,NORMAL,IND,10%
Model_46 I/O,3.3V,Pull-down,NORMAL,IND,10%
Model_47 I/O,3.3V,Pull-up,NORMAL,IND,10%
Model_48 I/O,3.3V,Pull-up/down off,NORMAL,IND,10%
|   Usage I/O#1.8/3.3#X#X#BI2C1833DVFZP18_SSDHH.PAD
|   Base model BI2C1833DVFZP18_SSDHH
[Model Selector] Selector_2
Model_65 I/O_OPEN_DRAIN,1.8V,NORMAL,I2C STANDARD,IND,5%
Model_66 I/O_OPEN_DRAIN,3.3V,NORMAL,I2C STANDARD,IND,5%
Model_67 I/O_OPEN_DRAIN,1.8V,NORMAL,I2C STANDARD,IND,10%
Model_68 I/O_OPEN_DRAIN,3.3V,NORMAL,I2C STANDARD,IND,10%
|   Usage INPUT#1.8/3.3#X#X#BC1833DV50BPBFBP18LL_SSDHV.PAD
|   Base model BC1833DV50BPBFBP18LL_SSDHV
[Model Selector] Selector_3
Model_37 I/O,1.8V,Pull-down,NORMAL,IND,5%
Model_38 I/O,1.8V,Pull-up,NORMAL,IND,5%
Model_39 I/O,1.8V,Pull-up/down off,NORMAL,IND,5%
Model_40 I/O,3.3V,Pull-down,NORMAL,IND,5%
Model_41 I/O,3.3V,Pull-up,NORMAL,IND,5%
Model_42 I/O,3.3V,Pull-up/down off,NORMAL,IND,5%
Model_43 I/O,1.8V,Pull-down,NORMAL,IND,10%
Model_44 I/O,1.8V,Pull-up,NORMAL,IND,10%
Model_45 I/O,1.8V,Pull-up/down off,NORMAL,IND,10%
Model_46 I/O,3.3V,Pull-down,NORMAL,IND,10%
Model_47 I/O,3.3V,Pull-up,NORMAL,IND,10%
Model_48 I/O,3.3V,Pull-up/down off,NORMAL,IND,10%
|   Usage OUTPUT#1.8/3.3#X#X#BC1833DV40DCPBFBP18LL_SSDHH.PAD
|   Base model BC1833DV40DCPBFBP18LL_SSDHH
[Model Selector] Selector_4
Model_1 I/O,1.8V,Pull-up/down off,slow,IND,5%
Model_10 I/O,3.3V,Pull-up,fast,IND,5%
Model_11 I/O,3.3V,Pull-up/down off,fast,IND,5%
Model_12 I/O,3.3V,Pull-up,slow,IND,5%
Model_13 I/O,1.8V,Pull-up/down off,slow,IND,10%
Model_14 I/O,1.8V,Pull-down,fast,IND,10%
Model_15 I/O,1.8V,Pull-down,slow,IND,10%
Model_16 I/O,1.8V,Pull-up,fast,IND,10%
Model_17 I/O,1.8V,Pull-up/down off,fast,IND,10%
Model_18 I/O,1.8V,Pull-up,slow,IND,10%
Model_19 I/O,3.3V,Pull-up/down off,slow,IND,10%
Model_2 I/O,1.8V,Pull-down,fast,IND,5%
Model_20 I/O,3.3V,Pull-down,fast,IND,10%
Model_21 I/O,3.3V,Pull-down,slow,IND,10%
Model_22 I/O,3.3V,Pull-up,fast,IND,10%
Model_23 I/O,3.3V,Pull-up/down off,fast,IND,10%
Model_24 I/O,3.3V,Pull-up,slow,IND,10%
Model_3 I/O,1.8V,Pull-down,slow,IND,5%
Model_4 I/O,1.8V,Pull-up,fast,IND,5%
Model_5 I/O,1.8V,Pull-up/down off,fast,IND,5%
Model_6 I/O,1.8V,Pull-up,slow,IND,5%
Model_7 I/O,3.3V,Pull-up/down off,slow,IND,5%
Model_8 I/O,3.3V,Pull-down,fast,IND,5%
Model_9 I/O,3.3V,Pull-down,slow,IND,5%
|   Usage I/O#1.8/3.3#X#X#BC1833DV40DCPBFBP18LL_SSDHH.PAD
|   Base model BC1833DV40DCPBFBP18LL_SSDHH
[Model Selector] Selector_5
Model_1 I/O,1.8V,Pull-up/down off,slow,IND,5%
Model_10 I/O,3.3V,Pull-up,fast,IND,5%
Model_11 I/O,3.3V,Pull-up/down off,fast,IND,5%
Model_12 I/O,3.3V,Pull-up,slow,IND,5%
Model_13 I/O,1.8V,Pull-up/down off,slow,IND,10%
Model_14 I/O,1.8V,Pull-down,fast,IND,10%
Model_15 I/O,1.8V,Pull-down,slow,IND,10%
Model_16 I/O,1.8V,Pull-up,fast,IND,10%
Model_17 I/O,1.8V,Pull-up/down off,fast,IND,10%
Model_18 I/O,1.8V,Pull-up,slow,IND,10%
Model_19 I/O,3.3V,Pull-up/down off,slow,IND,10%
Model_2 I/O,1.8V,Pull-down,fast,IND,5%
Model_20 I/O,3.3V,Pull-down,fast,IND,10%
Model_21 I/O,3.3V,Pull-down,slow,IND,10%
Model_22 I/O,3.3V,Pull-up,fast,IND,10%
Model_23 I/O,3.3V,Pull-up/down off,fast,IND,10%
Model_24 I/O,3.3V,Pull-up,slow,IND,10%
Model_3 I/O,1.8V,Pull-down,slow,IND,5%
Model_4 I/O,1.8V,Pull-up,fast,IND,5%
Model_5 I/O,1.8V,Pull-up/down off,fast,IND,5%
Model_6 I/O,1.8V,Pull-up,slow,IND,5%
Model_7 I/O,3.3V,Pull-up/down off,slow,IND,5%
Model_8 I/O,3.3V,Pull-down,fast,IND,5%
Model_9 I/O,3.3V,Pull-down,slow,IND,5%
|   Usage INPUT#1.8/3.3#X#X#IHHV1833DVHYP18LL_SSDHH.PAD
|   Base model IHHV1833DVHYP18LL_SSDHH
[Model Selector] Selector_6
Model_49 INPUT,1.8V,NORMAL,IND,5%
Model_50 INPUT,3.3V,NORMAL,IND,5%
Model_51 INPUT,1.8V,NORMAL,IND,10%
Model_52 INPUT,3.3V,NORMAL,IND,10%
|   Usage INPUT#1.8/3.3#X#X#BC1833DV50BPBFBP18LL_SSDHH.PAD
|   Base model BC1833DV50BPBFBP18LL_SSDHH
[Model Selector] Selector_7
Model_53 I/O,1.8V,Pull-down,NORMAL,IND,5%
Model_54 I/O,1.8V,Pull-up,NORMAL,IND,5%
Model_55 I/O,1.8V,Pull-up/down off,NORMAL,IND,5%
Model_56 I/O,3.3V,Pull-down,NORMAL,IND,5%
Model_57 I/O,3.3V,Pull-up,NORMAL,IND,5%
Model_58 I/O,3.3V,Pull-up/down off,NORMAL,IND,5%
Model_59 I/O,1.8V,Pull-down,NORMAL,IND,10%
Model_60 I/O,1.8V,Pull-up,NORMAL,IND,10%
Model_61 I/O,1.8V,Pull-up/down off,NORMAL,IND,10%
Model_62 I/O,3.3V,Pull-down,NORMAL,IND,10%
Model_63 I/O,3.3V,Pull-up,NORMAL,IND,10%
Model_64 I/O,3.3V,Pull-up/down off,NORMAL,IND,10%
|   Usage I/O#1.5/1.8#X#X#BCSHTLTCSCDVPBFZ_SSDHV.PAD
|   Base model BCSHTLTCSCDVPBFZ_SSDHV
[Model Selector] Selector_8
Model_100 3-STATE,1.8V,ODT off,slow, 0.67*RExt,IND,5%
Model_101 3-STATE,1.5V,ODT off,slowest, 1.00*RExt,IND,10%
Model_102 3-STATE,1.5V,ODT off,slowest, 1.60*RExt,IND,10%
Model_103 3-STATE,1.5V,ODT off,slow, 1.14*RExt,IND,10%
Model_104 3-STATE,1.5V,ODT off,slow, 1.33*RExt,IND,10%
Model_105 3-STATE,1.5V,ODT off,slowest, 0.88*RExt,IND,10%
Model_106 3-STATE,1.5V,ODT off,slow, 0.73*RExt,IND,10%
Model_107 3-STATE,1.5V,ODT off,slowest, 0.67*RExt,IND,10%
Model_108 3-STATE,1.5V,ODT off,slowest, 1.14*RExt,IND,10%
Model_109 3-STATE,1.5V,ODT off,slow, 0.80*RExt,IND,10%
Model_110 3-STATE,1.5V,ODT off,slowest, 1.33*RExt,IND,10%
Model_111 3-STATE,1.5V,ODT off,slow, 1.00*RExt,IND,10%
Model_112 3-STATE,1.5V,ODT off,slow, 1.60*RExt,IND,10%
Model_113 3-STATE,1.5V,ODT off,slowest, 0.73*RExt,IND,10%
Model_114 3-STATE,1.5V,ODT off,slowest, 0.80*RExt,IND,10%
Model_115 3-STATE,1.5V,ODT off,slow, 0.88*RExt,IND,10%
Model_116 3-STATE,1.5V,ODT off,slow, 0.67*RExt,IND,10%
Model_117 3-STATE,1.5V,ODT off,slowest, 1.00*RExt,IND,5%
Model_118 3-STATE,1.5V,ODT off,slowest, 1.60*RExt,IND,5%
Model_119 3-STATE,1.5V,ODT off,slow, 1.14*RExt,IND,5%
Model_120 3-STATE,1.5V,ODT off,slow, 1.33*RExt,IND,5%
Model_121 3-STATE,1.5V,ODT off,slowest, 0.88*RExt,IND,5%
Model_122 3-STATE,1.5V,ODT off,slow, 0.73*RExt,IND,5%
Model_123 3-STATE,1.5V,ODT off,slowest, 0.67*RExt,IND,5%
Model_124 3-STATE,1.5V,ODT off,slowest, 1.14*RExt,IND,5%
Model_125 3-STATE,1.5V,ODT off,slow, 0.80*RExt,IND,5%
Model_126 3-STATE,1.5V,ODT off,slowest, 1.33*RExt,IND,5%
Model_127 3-STATE,1.5V,ODT off,slow, 1.00*RExt,IND,5%
Model_128 3-STATE,1.5V,ODT off,slow, 1.60*RExt,IND,5%
Model_129 3-STATE,1.5V,ODT off,slowest, 0.73*RExt,IND,5%
Model_130 3-STATE,1.5V,ODT off,slowest, 0.80*RExt,IND,5%
Model_131 3-STATE,1.5V,ODT off,slow, 0.88*RExt,IND,5%
Model_132 3-STATE,1.5V,ODT off,slow, 0.67*RExt,IND,5%
Model_133 3-STATE,1.8V,ODT off,fast, 0.67*RExt,IND,10%
Model_134 3-STATE,1.8V,ODT off,fastest, 1.60*RExt,IND,10%
Model_135 3-STATE,1.8V,ODT off,fastest, 0.88*RExt,IND,10%
Model_136 3-STATE,1.8V,ODT off,fast, 1.60*RExt,IND,10%
Model_137 3-STATE,1.8V,ODT off,fastest, 1.14*RExt,IND,10%
Model_138 3-STATE,1.8V,ODT off,fastest, 1.33*RExt,IND,10%
Model_139 3-STATE,1.8V,ODT off,fast, 0.88*RExt,IND,10%
Model_140 3-STATE,1.8V,ODT off,fastest, 0.73*RExt,IND,10%
Model_141 3-STATE,1.8V,ODT off,fast, 1.14*RExt,IND,10%
Model_142 3-STATE,1.8V,ODT off,fastest, 0.80*RExt,IND,10%
Model_143 3-STATE,1.8V,ODT off,fast, 1.33*RExt,IND,10%
Model_144 3-STATE,1.8V,ODT off,fastest, 1.00*RExt,IND,10%
Model_145 3-STATE,1.8V,ODT off,fast, 0.73*RExt,IND,10%
Model_146 3-STATE,1.8V,ODT off,fast, 0.80*RExt,IND,10%
Model_147 3-STATE,1.8V,ODT off,fastest, 0.67*RExt,IND,10%
Model_148 3-STATE,1.8V,ODT off,fast, 1.00*RExt,IND,10%
Model_149 3-STATE,1.8V,ODT off,fast, 0.67*RExt,IND,5%
Model_150 3-STATE,1.8V,ODT off,fastest, 1.60*RExt,IND,5%
Model_151 3-STATE,1.8V,ODT off,fastest, 0.88*RExt,IND,5%
Model_152 3-STATE,1.8V,ODT off,fast, 1.60*RExt,IND,5%
Model_153 3-STATE,1.8V,ODT off,fastest, 1.14*RExt,IND,5%
Model_154 3-STATE,1.8V,ODT off,fastest, 1.33*RExt,IND,5%
Model_155 3-STATE,1.8V,ODT off,fast, 0.88*RExt,IND,5%
Model_156 3-STATE,1.8V,ODT off,fastest, 0.73*RExt,IND,5%
Model_157 3-STATE,1.8V,ODT off,fast, 1.14*RExt,IND,5%
Model_158 3-STATE,1.8V,ODT off,fastest, 0.80*RExt,IND,5%
Model_159 3-STATE,1.8V,ODT off,fast, 1.33*RExt,IND,5%
Model_160 3-STATE,1.8V,ODT off,fastest, 1.00*RExt,IND,5%
Model_161 3-STATE,1.8V,ODT off,fast, 0.73*RExt,IND,5%
Model_162 3-STATE,1.8V,ODT off,fast, 0.80*RExt,IND,5%
Model_163 3-STATE,1.8V,ODT off,fastest, 0.67*RExt,IND,5%
Model_164 3-STATE,1.8V,ODT off,fast, 1.00*RExt,IND,5%
Model_165 3-STATE,1.5V,ODT off,fast, 0.67*RExt,IND,10%
Model_166 3-STATE,1.5V,ODT off,fastest, 1.60*RExt,IND,10%
Model_167 3-STATE,1.5V,ODT off,fastest, 0.88*RExt,IND,10%
Model_168 3-STATE,1.5V,ODT off,fast, 1.60*RExt,IND,10%
Model_169 3-STATE,1.5V,ODT off,fastest, 1.14*RExt,IND,10%
Model_170 3-STATE,1.5V,ODT off,fastest, 1.33*RExt,IND,10%
Model_171 3-STATE,1.5V,ODT off,fast, 0.88*RExt,IND,10%
Model_172 3-STATE,1.5V,ODT off,fastest, 0.73*RExt,IND,10%
Model_173 3-STATE,1.5V,ODT off,fast, 1.14*RExt,IND,10%
Model_174 3-STATE,1.5V,ODT off,fastest, 0.80*RExt,IND,10%
Model_175 3-STATE,1.5V,ODT off,fast, 1.33*RExt,IND,10%
Model_176 3-STATE,1.5V,ODT off,fastest, 1.00*RExt,IND,10%
Model_177 3-STATE,1.5V,ODT off,fast, 0.73*RExt,IND,10%
Model_178 3-STATE,1.5V,ODT off,fast, 0.80*RExt,IND,10%
Model_179 3-STATE,1.5V,ODT off,fastest, 0.67*RExt,IND,10%
Model_180 3-STATE,1.5V,ODT off,fast, 1.00*RExt,IND,10%
Model_181 3-STATE,1.5V,ODT off,fast, 0.67*RExt,IND,5%
Model_182 3-STATE,1.5V,ODT off,fastest, 1.60*RExt,IND,5%
Model_183 3-STATE,1.5V,ODT off,fastest, 0.88*RExt,IND,5%
Model_184 3-STATE,1.5V,ODT off,fast, 1.60*RExt,IND,5%
Model_185 3-STATE,1.5V,ODT off,fastest, 1.14*RExt,IND,5%
Model_186 3-STATE,1.5V,ODT off,fastest, 1.33*RExt,IND,5%
Model_187 3-STATE,1.5V,ODT off,fast, 0.88*RExt,IND,5%
Model_188 3-STATE,1.5V,ODT off,fastest, 0.73*RExt,IND,5%
Model_189 3-STATE,1.5V,ODT off,fast, 1.14*RExt,IND,5%
Model_190 3-STATE,1.5V,ODT off,fastest, 0.80*RExt,IND,5%
Model_191 3-STATE,1.5V,ODT off,fast, 1.33*RExt,IND,5%
Model_192 3-STATE,1.5V,ODT off,fastest, 1.00*RExt,IND,5%
Model_193 3-STATE,1.5V,ODT off,fast, 0.73*RExt,IND,5%
Model_194 3-STATE,1.5V,ODT off,fast, 0.80*RExt,IND,5%
Model_195 3-STATE,1.5V,ODT off,fastest, 0.67*RExt,IND,5%
Model_196 3-STATE,1.5V,ODT off,fast, 1.00*RExt,IND,5%
Model_197 INPUT,1.8V,Half Thevenin, 0.67*RExt,IND,10%
Model_198 INPUT,1.8V,Pull-up/down off,IND,10%
Model_199 INPUT,1.8V,Pull-down,IND,10%
Model_200 INPUT,1.8V,FULLTERM, 1.60*RExt,IND,10%
Model_201 INPUT,1.8V,Half Thevenin, 1.60*RExt,IND,10%
Model_202 INPUT,1.8V,Pull-up,IND,10%
Model_203 INPUT,1.8V,FULLTERM, 0.88*RExt,IND,10%
Model_204 INPUT,1.8V,FULLTERM, 1.14*RExt,IND,10%
Model_205 INPUT,1.8V,Half Thevenin, 0.88*RExt,IND,10%
Model_206 INPUT,1.8V,FULLTERM, 1.33*RExt,IND,10%
Model_207 INPUT,1.8V,Half Thevenin, 1.14*RExt,IND,10%
Model_208 INPUT,1.8V,Half Thevenin, 1.33*RExt,IND,10%
Model_209 INPUT,1.8V,FULLTERM, 0.73*RExt,IND,10%
Model_210 INPUT,1.8V,Pull-up/down off,IND,10%
Model_211 INPUT,1.8V,FULLTERM, 0.80*RExt,IND,10%
Model_212 INPUT,1.8V,Half Thevenin, 0.73*RExt,IND,10%
Model_213 INPUT,1.8V,FULLTERM, 1.00*RExt,IND,10%
Model_214 INPUT,1.8V,Half Thevenin, 0.80*RExt,IND,10%
Model_215 INPUT,1.8V,Pull-down,IND,10%
Model_216 INPUT,1.8V,Half Thevenin, 1.00*RExt,IND,10%
Model_217 INPUT,1.8V,Pull-up,IND,10%
Model_218 INPUT,1.8V,FULLTERM, 0.67*RExt,IND,10%
Model_219 INPUT,1.8V,Half Thevenin, 0.67*RExt,IND,5%
Model_220 INPUT,1.8V,Pull-up/down off,IND,5%
Model_221 INPUT,1.8V,Pull-down,IND,5%
Model_222 INPUT,1.8V,FULLTERM, 1.60*RExt,IND,5%
Model_223 INPUT,1.8V,Half Thevenin, 1.60*RExt,IND,5%
Model_224 INPUT,1.8V,Pull-up,IND,5%
Model_225 INPUT,1.8V,FULLTERM, 0.88*RExt,IND,5%
Model_226 INPUT,1.8V,FULLTERM, 1.14*RExt,IND,5%
Model_227 INPUT,1.8V,Half Thevenin, 0.88*RExt,IND,5%
Model_228 INPUT,1.8V,FULLTERM, 1.33*RExt,IND,5%
Model_229 INPUT,1.8V,Half Thevenin, 1.14*RExt,IND,5%
Model_230 INPUT,1.8V,Half Thevenin, 1.33*RExt,IND,5%
Model_231 INPUT,1.8V,FULLTERM, 0.73*RExt,IND,5%
Model_232 INPUT,1.8V,Pull-up/down off,IND,5%
Model_233 INPUT,1.8V,FULLTERM, 0.80*RExt,IND,5%
Model_234 INPUT,1.8V,Half Thevenin, 0.73*RExt,IND,5%
Model_235 INPUT,1.8V,FULLTERM, 1.00*RExt,IND,5%
Model_236 INPUT,1.8V,Half Thevenin, 0.80*RExt,IND,5%
Model_237 INPUT,1.8V,Pull-down,IND,5%
Model_238 INPUT,1.8V,Half Thevenin, 1.00*RExt,IND,5%
Model_239 INPUT,1.8V,Pull-up,IND,5%
Model_240 INPUT,1.8V,FULLTERM, 0.67*RExt,IND,5%
Model_241 INPUT,1.5V,FULLTERM, 1.14*RExt,IND,10%
Model_242 INPUT,1.5V,FULLTERM, 1.33*RExt,IND,10%
Model_243 INPUT,1.5V,Half Thevenin, 0.67*RExt,IND,10%
Model_244 INPUT,1.5V,FULLTERM, 1.60*RExt,IND,10%
Model_245 INPUT,1.5V,Pull-up,IND,10%
Model_246 INPUT,1.5V,Half Thevenin, 0.73*RExt,IND,10%
Model_247 INPUT,1.5V,Half Thevenin, 0.80*RExt,IND,10%
Model_248 INPUT,1.5V,Half Thevenin, 1.00*RExt,IND,10%
Model_249 INPUT,1.5V,FULLTERM, 0.67*RExt,IND,10%
Model_250 INPUT,1.5V,Half Thevenin, 0.88*RExt,IND,10%
Model_251 INPUT,1.5V,Pull-up/down off,IND,10%
Model_252 INPUT,1.5V,Half Thevenin, 1.14*RExt,IND,10%
Model_253 INPUT,1.5V,Half Thevenin, 1.33*RExt,IND,10%
Model_254 INPUT,1.5V,FULLTERM, 0.73*RExt,IND,10%
Model_255 INPUT,1.5V,FULLTERM, 0.80*RExt,IND,10%
Model_256 INPUT,1.5V,Pull-down,IND,10%
Model_257 INPUT,1.5V,FULLTERM, 1.00*RExt,IND,10%
Model_258 INPUT,1.5V,Half Thevenin, 1.60*RExt,IND,10%
Model_259 INPUT,1.5V,FULLTERM, 0.88*RExt,IND,10%
Model_260 INPUT,1.5V,FULLTERM, 1.14*RExt,IND,5%
Model_261 INPUT,1.5V,FULLTERM, 1.33*RExt,IND,5%
Model_262 INPUT,1.5V,Half Thevenin, 0.67*RExt,IND,5%
Model_263 INPUT,1.5V,FULLTERM, 1.60*RExt,IND,5%
Model_264 INPUT,1.5V,Pull-up,IND,5%
Model_265 INPUT,1.5V,Half Thevenin, 0.73*RExt,IND,5%
Model_266 INPUT,1.5V,Half Thevenin, 0.80*RExt,IND,5%
Model_267 INPUT,1.5V,Half Thevenin, 1.00*RExt,IND,5%
Model_268 INPUT,1.5V,FULLTERM, 0.67*RExt,IND,5%
Model_269 INPUT,1.5V,Half Thevenin, 0.88*RExt,IND,5%
Model_270 INPUT,1.5V,Pull-up/down off,IND,5%
Model_271 INPUT,1.5V,Half Thevenin, 1.14*RExt,IND,5%
Model_272 INPUT,1.5V,Half Thevenin, 1.33*RExt,IND,5%
Model_273 INPUT,1.5V,FULLTERM, 0.73*RExt,IND,5%
Model_274 INPUT,1.5V,FULLTERM, 0.80*RExt,IND,5%
Model_275 INPUT,1.5V,Pull-down,IND,5%
Model_276 INPUT,1.5V,FULLTERM, 1.00*RExt,IND,5%
Model_277 INPUT,1.5V,Half Thevenin, 1.60*RExt,IND,5%
Model_278 INPUT,1.5V,FULLTERM, 0.88*RExt,IND,5%
Model_69 3-STATE,1.8V,ODT off,slowest, 1.00*RExt,IND,10%
Model_70 3-STATE,1.8V,ODT off,slowest, 1.60*RExt,IND,10%
Model_71 3-STATE,1.8V,ODT off,slow, 1.14*RExt,IND,10%
Model_72 3-STATE,1.8V,ODT off,slow, 1.33*RExt,IND,10%
Model_73 3-STATE,1.8V,ODT off,slowest, 0.88*RExt,IND,10%
Model_74 3-STATE,1.8V,ODT off,slow, 0.73*RExt,IND,10%
Model_75 3-STATE,1.8V,ODT off,slowest, 0.67*RExt,IND,10%
Model_76 3-STATE,1.8V,ODT off,slowest, 1.14*RExt,IND,10%
Model_77 3-STATE,1.8V,ODT off,slow, 0.80*RExt,IND,10%
Model_78 3-STATE,1.8V,ODT off,slowest, 1.33*RExt,IND,10%
Model_79 3-STATE,1.8V,ODT off,slow, 1.00*RExt,IND,10%
Model_80 3-STATE,1.8V,ODT off,slow, 1.60*RExt,IND,10%
Model_81 3-STATE,1.8V,ODT off,slowest, 0.73*RExt,IND,10%
Model_82 3-STATE,1.8V,ODT off,slowest, 0.80*RExt,IND,10%
Model_83 3-STATE,1.8V,ODT off,slow, 0.88*RExt,IND,10%
Model_84 3-STATE,1.8V,ODT off,slow, 0.67*RExt,IND,10%
Model_85 3-STATE,1.8V,ODT off,slowest, 1.00*RExt,IND,5%
Model_86 3-STATE,1.8V,ODT off,slowest, 1.60*RExt,IND,5%
Model_87 3-STATE,1.8V,ODT off,slow, 1.14*RExt,IND,5%
Model_88 3-STATE,1.8V,ODT off,slow, 1.33*RExt,IND,5%
Model_89 3-STATE,1.8V,ODT off,slowest, 0.88*RExt,IND,5%
Model_90 3-STATE,1.8V,ODT off,slow, 0.73*RExt,IND,5%
Model_91 3-STATE,1.8V,ODT off,slowest, 0.67*RExt,IND,5%
Model_92 3-STATE,1.8V,ODT off,slowest, 1.14*RExt,IND,5%
Model_93 3-STATE,1.8V,ODT off,slow, 0.80*RExt,IND,5%
Model_94 3-STATE,1.8V,ODT off,slowest, 1.33*RExt,IND,5%
Model_95 3-STATE,1.8V,ODT off,slow, 1.00*RExt,IND,5%
Model_96 3-STATE,1.8V,ODT off,slow, 1.60*RExt,IND,5%
Model_97 3-STATE,1.8V,ODT off,slowest, 0.73*RExt,IND,5%
Model_98 3-STATE,1.8V,ODT off,slowest, 0.80*RExt,IND,5%
Model_99 3-STATE,1.8V,ODT off,slow, 0.88*RExt,IND,5%
|   Usage OUTPUT#1.5/1.8#X#X#BCSHTLTCSCDVPBFZ_SSDHV.PAD
|   Base model BCSHTLTCSCDVPBFZ_SSDHV
[Model Selector] Selector_9
Model_100 3-STATE,1.8V,ODT off,slow, 0.67*RExt,IND,5%
Model_101 3-STATE,1.5V,ODT off,slowest, 1.00*RExt,IND,10%
Model_102 3-STATE,1.5V,ODT off,slowest, 1.60*RExt,IND,10%
Model_103 3-STATE,1.5V,ODT off,slow, 1.14*RExt,IND,10%
Model_104 3-STATE,1.5V,ODT off,slow, 1.33*RExt,IND,10%
Model_105 3-STATE,1.5V,ODT off,slowest, 0.88*RExt,IND,10%
Model_106 3-STATE,1.5V,ODT off,slow, 0.73*RExt,IND,10%
Model_107 3-STATE,1.5V,ODT off,slowest, 0.67*RExt,IND,10%
Model_108 3-STATE,1.5V,ODT off,slowest, 1.14*RExt,IND,10%
Model_109 3-STATE,1.5V,ODT off,slow, 0.80*RExt,IND,10%
Model_110 3-STATE,1.5V,ODT off,slowest, 1.33*RExt,IND,10%
Model_111 3-STATE,1.5V,ODT off,slow, 1.00*RExt,IND,10%
Model_112 3-STATE,1.5V,ODT off,slow, 1.60*RExt,IND,10%
Model_113 3-STATE,1.5V,ODT off,slowest, 0.73*RExt,IND,10%
Model_114 3-STATE,1.5V,ODT off,slowest, 0.80*RExt,IND,10%
Model_115 3-STATE,1.5V,ODT off,slow, 0.88*RExt,IND,10%
Model_116 3-STATE,1.5V,ODT off,slow, 0.67*RExt,IND,10%
Model_117 3-STATE,1.5V,ODT off,slowest, 1.00*RExt,IND,5%
Model_118 3-STATE,1.5V,ODT off,slowest, 1.60*RExt,IND,5%
Model_119 3-STATE,1.5V,ODT off,slow, 1.14*RExt,IND,5%
Model_120 3-STATE,1.5V,ODT off,slow, 1.33*RExt,IND,5%
Model_121 3-STATE,1.5V,ODT off,slowest, 0.88*RExt,IND,5%
Model_122 3-STATE,1.5V,ODT off,slow, 0.73*RExt,IND,5%
Model_123 3-STATE,1.5V,ODT off,slowest, 0.67*RExt,IND,5%
Model_124 3-STATE,1.5V,ODT off,slowest, 1.14*RExt,IND,5%
Model_125 3-STATE,1.5V,ODT off,slow, 0.80*RExt,IND,5%
Model_126 3-STATE,1.5V,ODT off,slowest, 1.33*RExt,IND,5%
Model_127 3-STATE,1.5V,ODT off,slow, 1.00*RExt,IND,5%
Model_128 3-STATE,1.5V,ODT off,slow, 1.60*RExt,IND,5%
Model_129 3-STATE,1.5V,ODT off,slowest, 0.73*RExt,IND,5%
Model_130 3-STATE,1.5V,ODT off,slowest, 0.80*RExt,IND,5%
Model_131 3-STATE,1.5V,ODT off,slow, 0.88*RExt,IND,5%
Model_132 3-STATE,1.5V,ODT off,slow, 0.67*RExt,IND,5%
Model_133 3-STATE,1.8V,ODT off,fast, 0.67*RExt,IND,10%
Model_134 3-STATE,1.8V,ODT off,fastest, 1.60*RExt,IND,10%
Model_135 3-STATE,1.8V,ODT off,fastest, 0.88*RExt,IND,10%
Model_136 3-STATE,1.8V,ODT off,fast, 1.60*RExt,IND,10%
Model_137 3-STATE,1.8V,ODT off,fastest, 1.14*RExt,IND,10%
Model_138 3-STATE,1.8V,ODT off,fastest, 1.33*RExt,IND,10%
Model_139 3-STATE,1.8V,ODT off,fast, 0.88*RExt,IND,10%
Model_140 3-STATE,1.8V,ODT off,fastest, 0.73*RExt,IND,10%
Model_141 3-STATE,1.8V,ODT off,fast, 1.14*RExt,IND,10%
Model_142 3-STATE,1.8V,ODT off,fastest, 0.80*RExt,IND,10%
Model_143 3-STATE,1.8V,ODT off,fast, 1.33*RExt,IND,10%
Model_144 3-STATE,1.8V,ODT off,fastest, 1.00*RExt,IND,10%
Model_145 3-STATE,1.8V,ODT off,fast, 0.73*RExt,IND,10%
Model_146 3-STATE,1.8V,ODT off,fast, 0.80*RExt,IND,10%
Model_147 3-STATE,1.8V,ODT off,fastest, 0.67*RExt,IND,10%
Model_148 3-STATE,1.8V,ODT off,fast, 1.00*RExt,IND,10%
Model_149 3-STATE,1.8V,ODT off,fast, 0.67*RExt,IND,5%
Model_150 3-STATE,1.8V,ODT off,fastest, 1.60*RExt,IND,5%
Model_151 3-STATE,1.8V,ODT off,fastest, 0.88*RExt,IND,5%
Model_152 3-STATE,1.8V,ODT off,fast, 1.60*RExt,IND,5%
Model_153 3-STATE,1.8V,ODT off,fastest, 1.14*RExt,IND,5%
Model_154 3-STATE,1.8V,ODT off,fastest, 1.33*RExt,IND,5%
Model_155 3-STATE,1.8V,ODT off,fast, 0.88*RExt,IND,5%
Model_156 3-STATE,1.8V,ODT off,fastest, 0.73*RExt,IND,5%
Model_157 3-STATE,1.8V,ODT off,fast, 1.14*RExt,IND,5%
Model_158 3-STATE,1.8V,ODT off,fastest, 0.80*RExt,IND,5%
Model_159 3-STATE,1.8V,ODT off,fast, 1.33*RExt,IND,5%
Model_160 3-STATE,1.8V,ODT off,fastest, 1.00*RExt,IND,5%
Model_161 3-STATE,1.8V,ODT off,fast, 0.73*RExt,IND,5%
Model_162 3-STATE,1.8V,ODT off,fast, 0.80*RExt,IND,5%
Model_163 3-STATE,1.8V,ODT off,fastest, 0.67*RExt,IND,5%
Model_164 3-STATE,1.8V,ODT off,fast, 1.00*RExt,IND,5%
Model_165 3-STATE,1.5V,ODT off,fast, 0.67*RExt,IND,10%
Model_166 3-STATE,1.5V,ODT off,fastest, 1.60*RExt,IND,10%
Model_167 3-STATE,1.5V,ODT off,fastest, 0.88*RExt,IND,10%
Model_168 3-STATE,1.5V,ODT off,fast, 1.60*RExt,IND,10%
Model_169 3-STATE,1.5V,ODT off,fastest, 1.14*RExt,IND,10%
Model_170 3-STATE,1.5V,ODT off,fastest, 1.33*RExt,IND,10%
Model_171 3-STATE,1.5V,ODT off,fast, 0.88*RExt,IND,10%
Model_172 3-STATE,1.5V,ODT off,fastest, 0.73*RExt,IND,10%
Model_173 3-STATE,1.5V,ODT off,fast, 1.14*RExt,IND,10%
Model_174 3-STATE,1.5V,ODT off,fastest, 0.80*RExt,IND,10%
Model_175 3-STATE,1.5V,ODT off,fast, 1.33*RExt,IND,10%
Model_176 3-STATE,1.5V,ODT off,fastest, 1.00*RExt,IND,10%
Model_177 3-STATE,1.5V,ODT off,fast, 0.73*RExt,IND,10%
Model_178 3-STATE,1.5V,ODT off,fast, 0.80*RExt,IND,10%
Model_179 3-STATE,1.5V,ODT off,fastest, 0.67*RExt,IND,10%
Model_180 3-STATE,1.5V,ODT off,fast, 1.00*RExt,IND,10%
Model_181 3-STATE,1.5V,ODT off,fast, 0.67*RExt,IND,5%
Model_182 3-STATE,1.5V,ODT off,fastest, 1.60*RExt,IND,5%
Model_183 3-STATE,1.5V,ODT off,fastest, 0.88*RExt,IND,5%
Model_184 3-STATE,1.5V,ODT off,fast, 1.60*RExt,IND,5%
Model_185 3-STATE,1.5V,ODT off,fastest, 1.14*RExt,IND,5%
Model_186 3-STATE,1.5V,ODT off,fastest, 1.33*RExt,IND,5%
Model_187 3-STATE,1.5V,ODT off,fast, 0.88*RExt,IND,5%
Model_188 3-STATE,1.5V,ODT off,fastest, 0.73*RExt,IND,5%
Model_189 3-STATE,1.5V,ODT off,fast, 1.14*RExt,IND,5%
Model_190 3-STATE,1.5V,ODT off,fastest, 0.80*RExt,IND,5%
Model_191 3-STATE,1.5V,ODT off,fast, 1.33*RExt,IND,5%
Model_192 3-STATE,1.5V,ODT off,fastest, 1.00*RExt,IND,5%
Model_193 3-STATE,1.5V,ODT off,fast, 0.73*RExt,IND,5%
Model_194 3-STATE,1.5V,ODT off,fast, 0.80*RExt,IND,5%
Model_195 3-STATE,1.5V,ODT off,fastest, 0.67*RExt,IND,5%
Model_196 3-STATE,1.5V,ODT off,fast, 1.00*RExt,IND,5%
Model_69 3-STATE,1.8V,ODT off,slowest, 1.00*RExt,IND,10%
Model_70 3-STATE,1.8V,ODT off,slowest, 1.60*RExt,IND,10%
Model_71 3-STATE,1.8V,ODT off,slow, 1.14*RExt,IND,10%
Model_72 3-STATE,1.8V,ODT off,slow, 1.33*RExt,IND,10%
Model_73 3-STATE,1.8V,ODT off,slowest, 0.88*RExt,IND,10%
Model_74 3-STATE,1.8V,ODT off,slow, 0.73*RExt,IND,10%
Model_75 3-STATE,1.8V,ODT off,slowest, 0.67*RExt,IND,10%
Model_76 3-STATE,1.8V,ODT off,slowest, 1.14*RExt,IND,10%
Model_77 3-STATE,1.8V,ODT off,slow, 0.80*RExt,IND,10%
Model_78 3-STATE,1.8V,ODT off,slowest, 1.33*RExt,IND,10%
Model_79 3-STATE,1.8V,ODT off,slow, 1.00*RExt,IND,10%
Model_80 3-STATE,1.8V,ODT off,slow, 1.60*RExt,IND,10%
Model_81 3-STATE,1.8V,ODT off,slowest, 0.73*RExt,IND,10%
Model_82 3-STATE,1.8V,ODT off,slowest, 0.80*RExt,IND,10%
Model_83 3-STATE,1.8V,ODT off,slow, 0.88*RExt,IND,10%
Model_84 3-STATE,1.8V,ODT off,slow, 0.67*RExt,IND,10%
Model_85 3-STATE,1.8V,ODT off,slowest, 1.00*RExt,IND,5%
Model_86 3-STATE,1.8V,ODT off,slowest, 1.60*RExt,IND,5%
Model_87 3-STATE,1.8V,ODT off,slow, 1.14*RExt,IND,5%
Model_88 3-STATE,1.8V,ODT off,slow, 1.33*RExt,IND,5%
Model_89 3-STATE,1.8V,ODT off,slowest, 0.88*RExt,IND,5%
Model_90 3-STATE,1.8V,ODT off,slow, 0.73*RExt,IND,5%
Model_91 3-STATE,1.8V,ODT off,slowest, 0.67*RExt,IND,5%
Model_92 3-STATE,1.8V,ODT off,slowest, 1.14*RExt,IND,5%
Model_93 3-STATE,1.8V,ODT off,slow, 0.80*RExt,IND,5%
Model_94 3-STATE,1.8V,ODT off,slowest, 1.33*RExt,IND,5%
Model_95 3-STATE,1.8V,ODT off,slow, 1.00*RExt,IND,5%
Model_96 3-STATE,1.8V,ODT off,slow, 1.60*RExt,IND,5%
Model_97 3-STATE,1.8V,ODT off,slowest, 0.73*RExt,IND,5%
Model_98 3-STATE,1.8V,ODT off,slowest, 0.80*RExt,IND,5%
Model_99 3-STATE,1.8V,ODT off,slow, 0.88*RExt,IND,5%
|   Usage OUTPUT#1.8/3.3#X#X#BC1833DV50BPBFBP18LL_SSDHH.PAD
|   Base model BC1833DV50BPBFBP18LL_SSDHH
[Model Selector] Selector_10
Model_53 I/O,1.8V,Pull-down,NORMAL,IND,5%
Model_54 I/O,1.8V,Pull-up,NORMAL,IND,5%
Model_55 I/O,1.8V,Pull-up/down off,NORMAL,IND,5%
Model_56 I/O,3.3V,Pull-down,NORMAL,IND,5%
Model_57 I/O,3.3V,Pull-up,NORMAL,IND,5%
Model_58 I/O,3.3V,Pull-up/down off,NORMAL,IND,5%
Model_59 I/O,1.8V,Pull-down,NORMAL,IND,10%
Model_60 I/O,1.8V,Pull-up,NORMAL,IND,10%
Model_61 I/O,1.8V,Pull-up/down off,NORMAL,IND,10%
Model_62 I/O,3.3V,Pull-down,NORMAL,IND,10%
Model_63 I/O,3.3V,Pull-up,NORMAL,IND,10%
Model_64 I/O,3.3V,Pull-up/down off,NORMAL,IND,10%
|   Usage I/O#1.8/3.3#X#X#BC1833DV50BPBFBP18LL_SSDHV.PAD
|   Base model BC1833DV50BPBFBP18LL_SSDHV
[Model Selector] Selector_11
Model_37 I/O,1.8V,Pull-down,NORMAL,IND,5%
Model_38 I/O,1.8V,Pull-up,NORMAL,IND,5%
Model_39 I/O,1.8V,Pull-up/down off,NORMAL,IND,5%
Model_40 I/O,3.3V,Pull-down,NORMAL,IND,5%
Model_41 I/O,3.3V,Pull-up,NORMAL,IND,5%
Model_42 I/O,3.3V,Pull-up/down off,NORMAL,IND,5%
Model_43 I/O,1.8V,Pull-down,NORMAL,IND,10%
Model_44 I/O,1.8V,Pull-up,NORMAL,IND,10%
Model_45 I/O,1.8V,Pull-up/down off,NORMAL,IND,10%
Model_46 I/O,3.3V,Pull-down,NORMAL,IND,10%
Model_47 I/O,3.3V,Pull-up,NORMAL,IND,10%
Model_48 I/O,3.3V,Pull-up/down off,NORMAL,IND,10%
|   Usage I/O#1.5/1.8#X#X#BCSHTLTCSCDDVPBFZ_SSDHV.PAD
|   Base model BCSHTLTCSCDDVPBFZ_SSDHV
[Model Selector] Selector_12
Model_279 3-STATE,1.8V,ODT off,slowest, 1.00*RExt,IND,10%
Model_280 3-STATE,1.8V,ODT off,slowest, 1.60*RExt,IND,10%
Model_281 3-STATE,1.8V,ODT off,slow, 1.14*RExt,IND,10%
Model_282 3-STATE,1.8V,ODT off,slow, 1.33*RExt,IND,10%
Model_283 3-STATE,1.8V,ODT off,slowest, 0.88*RExt,IND,10%
Model_284 3-STATE,1.8V,ODT off,slow, 0.73*RExt,IND,10%
Model_285 3-STATE,1.8V,ODT off,slowest, 0.67*RExt,IND,10%
Model_286 3-STATE,1.8V,ODT off,slowest, 1.14*RExt,IND,10%
Model_287 3-STATE,1.8V,ODT off,slow, 0.80*RExt,IND,10%
Model_288 3-STATE,1.8V,ODT off,slowest, 1.33*RExt,IND,10%
Model_289 3-STATE,1.8V,ODT off,slow, 1.00*RExt,IND,10%
Model_290 3-STATE,1.8V,ODT off,slow, 1.60*RExt,IND,10%
Model_291 3-STATE,1.8V,ODT off,slowest, 0.73*RExt,IND,10%
Model_292 3-STATE,1.8V,ODT off,slowest, 0.80*RExt,IND,10%
Model_293 3-STATE,1.8V,ODT off,slow, 0.88*RExt,IND,10%
Model_294 3-STATE,1.8V,ODT off,slow, 0.67*RExt,IND,10%
Model_295 3-STATE,1.8V,ODT off,slowest, 1.00*RExt,IND,5%
Model_296 3-STATE,1.8V,ODT off,slowest, 1.60*RExt,IND,5%
Model_297 3-STATE,1.8V,ODT off,slow, 1.14*RExt,IND,5%
Model_298 3-STATE,1.8V,ODT off,slow, 1.33*RExt,IND,5%
Model_299 3-STATE,1.8V,ODT off,slowest, 0.88*RExt,IND,5%
Model_300 3-STATE,1.8V,ODT off,slow, 0.73*RExt,IND,5%
Model_301 3-STATE,1.8V,ODT off,slowest, 0.67*RExt,IND,5%
Model_302 3-STATE,1.8V,ODT off,slowest, 1.14*RExt,IND,5%
Model_303 3-STATE,1.8V,ODT off,slow, 0.80*RExt,IND,5%
Model_304 3-STATE,1.8V,ODT off,slowest, 1.33*RExt,IND,5%
Model_305 3-STATE,1.8V,ODT off,slow, 1.00*RExt,IND,5%
Model_306 3-STATE,1.8V,ODT off,slow, 1.60*RExt,IND,5%
Model_307 3-STATE,1.8V,ODT off,slowest, 0.73*RExt,IND,5%
Model_308 3-STATE,1.8V,ODT off,slowest, 0.80*RExt,IND,5%
Model_309 3-STATE,1.8V,ODT off,slow, 0.88*RExt,IND,5%
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| Models and submodels in the file (640): Model_1 (I/O), Model_2 (I/O), Model_3 (I/O), Model_4 (I/O), Model_5 (I/O), Model_6 (I/O), Model_7 (I/O), Model_8 (I/O), Model_9 (I/O), Model_10 (I/O), Model_11 (I/O), Model_12 (I/O), Model_13 (I/O), Model_14 (I/O), Model_15 (I/O), Model_16 (I/O), Model_17 (I/O), Model_18 (I/O), Model_19 (I/O), Model_20 (I/O), Model_21 (I/O), Model_22 (I/O), Model_23 (I/O), Model_24 (I/O), Model_25 (Input), Model_26 (Input), Model_27 (Input), Model_28 (Input), Model_29 (Input), Model_30 (Input), Model_31 (Input), Model_32 (Input), Model_33 (Input), Model_34 (Input), Model_35 (Input), Model_36 (Input), Model_37 (I/O), Model_38 (I/O), Model_39 (I/O), Model_40 (I/O), Model_41 (I/O), Model_42 (I/O), Model_43 (I/O), Model_44 (I/O), Model_45 (I/O), Model_46 (I/O), Model_47 (I/O), Model_48 (I/O), Model_49 (Input), Model_50 (Input), Model_51 (Input), Model_52 (Input), Model_53 (I/O), Model_54 (I/O), Model_55 (I/O), Model_56 (I/O), Model_57 (I/O), Model_58 (I/O), Model_59 (I/O), Model_60 (I/O), Model_61 (I/O), Model_62 (I/O), Model_63 (I/O), Model_64 (I/O), Model_65 (I/O_open_drain), Model_66 (I/O_open_drain), Model_67 (I/O_open_drain), Model_68 (I/O_open_drain), Model_69 (3-state), Model_70 (3-state), Model_71 (3-state), Model_72 (3-state), Model_73 (3-state), Model_74 (3-state), Model_75 (3-state), Model_76 (3-state), Model_77 (3-state), Model_78 (3-state), Model_79 (3-state), Model_80 (3-state)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
